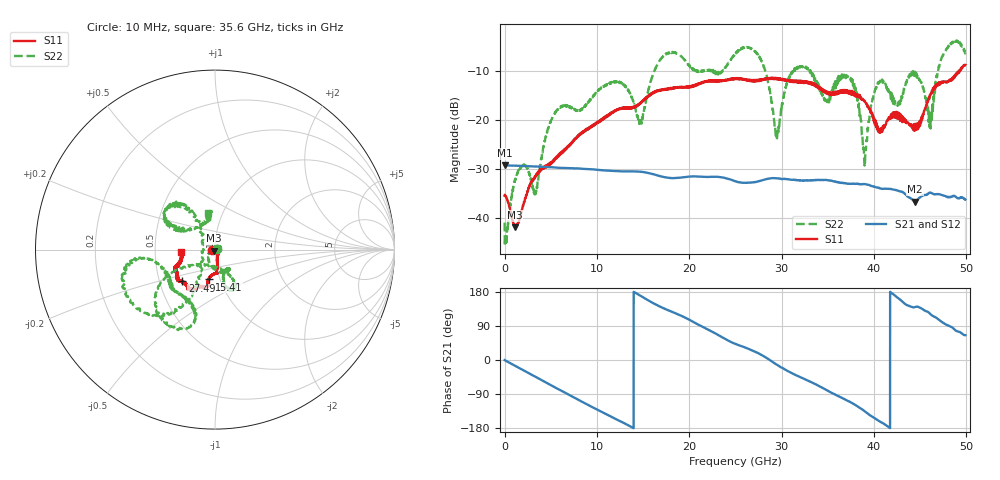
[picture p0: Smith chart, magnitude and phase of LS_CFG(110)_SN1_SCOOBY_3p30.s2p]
!Keysight Technologies,N5245B,MY58422026,A.13.80.08
!Date: Friday, March 20, 2020 00:01:42
!Correction: S11(Full 2 Port(1,2))
!S21(Full 2 Port(1,2))
!S12(Full 2 Port(1,2))
!S22(Full 2 Port(1,2))
!S2P File: Measurements: S11, S21, S12, S22:
# Hz S DB R 50.0
!freq dBS11 angS11 dBS21 angS21 dBS12 angS12 dBS22 angS22
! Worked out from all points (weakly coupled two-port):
!   4991 points, 10 MHz to 49.91 GHz, reference 50 ohm
!   highest |S21| = -29.27 dB at 10 MHz (marker M1); lowest = -36.7 dB at 44.45 GHz (marker M2)
!   lowest |S11| = -41.9 dB at 1.11 GHz (marker M3), VSWR 1.02, Z = 49.4 - j0.507 ohm
!   |S11| at or under -10 dB: start of sweep to 49.24 GHz; 49.30667 GHz to 49.32497 GHz (18.3 MHz wide, 0.0371 % of centre)
!   |S22| runs from -45.8 to -3.7 dB; largest |S21 - S12| = 0.00035
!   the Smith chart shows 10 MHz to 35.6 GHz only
!   S11 on the Smith chart (normalised r, x): 10 MHz: 0.97, -0.01; 15.41 GHz: 0.89, -0.30; 27.49 GHz: 0.66, -0.25; 35.6 GHz: 0.68, -0.02
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1e7  -35.49 -170.5  -29.27 -0.3  -29.25 -0.2  -41.03 6.1
1.11e9  -41.94 -140.0  -29.35 -14.9  -29.34 -14.8  -32.63 -26.8
3.32e9  -31.44 -59.9  -29.52 -43.9  -29.51 -43.9  -34.58 130.6
5.38e9  -28.03 -67.3  -29.71 -71.1  -29.70 -71.1  -18.85 -88.1
8.33e9  -22.83 -79.6  -29.97 -109.4  -29.96 -109.4  -17.81 -63.5
1.541e10  -15.41 -101.0  -30.78 159.7  -30.78 159.8  -15.37 -146.8
1.665e10  -14.03 -101.5  -31.39 143.1  -31.38 143.1  -8.28 -145.5
1.985e10  -13.22 -107.4  -31.63 108.3  -31.62 108.4  -8.60 -106.3
2.496e10  -11.59 -124.6  -32.49 42.7  -32.47 42.9  -6.55 -170.9
2.749e10  -11.92 -135.7  -32.57 17.8  -32.58 18.0  -6.66 -127.8
2.947e10  -11.40 -140.9  -31.94 -12.1  -31.93 -11.7  -23.32 -175.7
3.103e10  -11.95 -147.8  -32.22 -33.8  -32.24 -33.5  -10.39 125.8
3.328e10  -12.51 -157.9  -32.33 -59.4  -32.34 -58.9  -10.61 153.1
3.56e10  -14.35 -175.2  -32.57 -88.9  -32.51 -88.4  -13.90 101.4
3.77e10  -14.86 174.7  -33.05 -114.6  -32.99 -114.7  -12.17 131.6
3.902e10  -16.17 172.4  -33.12 -135.5  -33.09 -135.7  -28.53 -113.8
4.021e10  -21.21 161.3  -33.75 -155.7  -33.74 -155.9  -13.45 -8.7
4.16e10  -19.55 105.6  -34.11 -177.1  -34.13 -177.1  -14.13 22.5
4.445e10  -21.35 53.2  -36.71 139.8  -36.71 140.0  -10.37 -17.0
4.614e10  -14.75 6.9  -34.88 120.7  -34.89 121.0  -21.42 -50.7
4.757e10  -12.13 6.9  -35.49 97.1  -35.52 97.2  -6.27 -80.3
4.991e10  -8.70 -12.7  -36.29 65.4  -36.29 65.5  -6.27 -28.6
